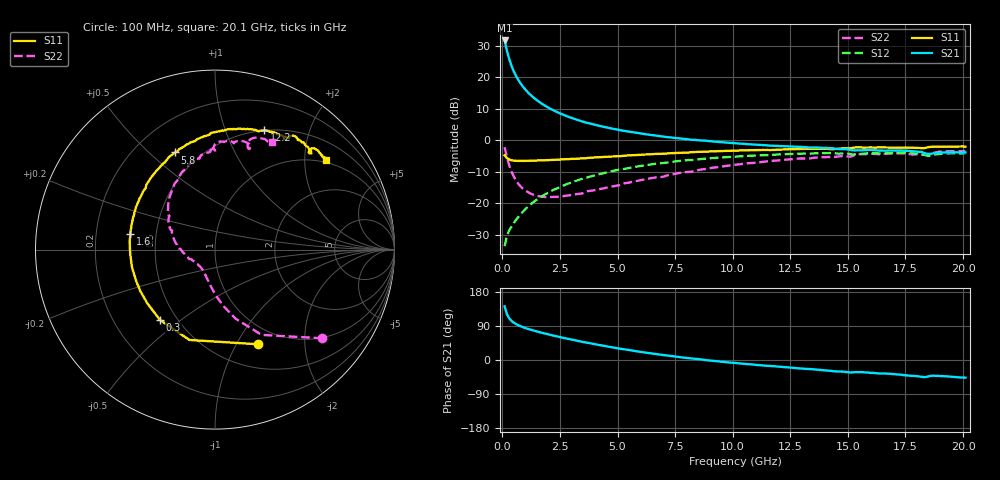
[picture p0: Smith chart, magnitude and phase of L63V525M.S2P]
!  Infineon Technologies AG
! BFR380L3 , PF131585-7, No.6, Th 09.10.01, soldered on pcb-board, measured with PP GSG850
!  Vce=3.5 V,  Ic=25.0 mA
! Common Emitter S-Parameters:  15. November 2001
#  GHz  S  MA  R  50
! f  S11  S21  S12  S22
! GHz  Mag  Ang  Mag  Ang  Mag  Ang  Mag  Ang
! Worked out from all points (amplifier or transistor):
!   201 points, 100 MHz to 20.1 GHz, reference 50 ohm
!   highest |S21| = 31.7 dB at 100 MHz (marker M1)
!   |S21| within 3 dB of that: start of sweep to 192.9 MHz
!   unconditionally stable (mu >= 1): 1.322 GHz to 4.375 GHz
!   at 3.4 GHz: K = 1.02, MAG = 8.4 dB, |S12| = -12.4 dB
!   at 10.1 GHz: K = 0.95, MSG = 2.1 dB, |S12| = -5.2 dB
!   at 20.1 GHz: K = 0.98, MSG = 0.1 dB, |S12| = -4.1 dB
!   S11 on the Smith chart (normalised r, x): 100 MHz: 0.77, -1.23; 300 MHz: 0.40, -0.42; 1.6 GHz: 0.35, +0.08; 5.8 GHz: 0.37, +0.61; 12.2 GHz: 0.50, +1.37; 20.1 GHz: 0.93, +2.52
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0.1  0.5786 -65.7  38.56 141.6  0.02089 64.5  0.7758 -39.6
0.2  0.5231 -105.8  26.59 120.9  0.03038 56.3  0.5417 -61.3
0.3  0.4978 -128.0  19.49 110.0  0.03731 55.2  0.4017 -73.4
0.4  0.4814 -141.8  15.2 103.2  0.04277 56.8  0.3181 -81.5
0.5  0.4759 -151.1  12.4 98.3  0.04872 58.8  0.2653 -87.6
0.6  0.473 -158.1  10.45 94.7  0.05495 60.4  0.2295 -92.4
0.7  0.4713 -163.8  9.031 91.6  0.06115 61.8  0.2036 -96.8
0.8  0.473 -168.0  7.943 88.9  0.06783 63.0  0.1847 -100.6
0.9  0.4714 -172.0  7.089 86.5  0.07415 63.6  0.1702 -104.1
1.1  0.4734 -178.3  5.848 82.4  0.08767 64.7  0.1515 -110.6
1.3  0.476 176.2  4.976 78.7  0.101 65.1  0.1393 -116.3
1.6  0.4796 169.5  4.079 73.6  0.1213 65.0  0.1296 -123.9
2  0.4861 161.7  3.301 67.5  0.1484 63.8  0.1256 -132.9
2.4  0.4945 155.1  2.787 61.8  0.1754 62.1  0.1266 -141.1
3.5  0.5157 138.8  1.979 47.6  0.2476 55.9  0.1448 -158.4
5.8  0.5851 112.3  1.322 23.3  0.381 40.7  0.226 169.1
6.8  0.6123 102.8  1.172 14.5  0.4321 33.5  0.2613 156.8
10.1  0.6877 78.4  0.9011 -7.7  0.5524 12.1  0.409 125.9
12.2  0.7195 67.6  0.8118 -18.7  0.603 -0.7  0.49 108.3
13.5  0.7331 61.1  0.7712 -24.6  0.62 -8.5  0.5259 99.0
16.8  0.7691 48.7  0.6899 -36.2  0.6283 -24.5  0.6177 78.1
20.1  0.7943 39.0  0.6442 -46.6  0.6232 -38.2  0.6763 62.0
